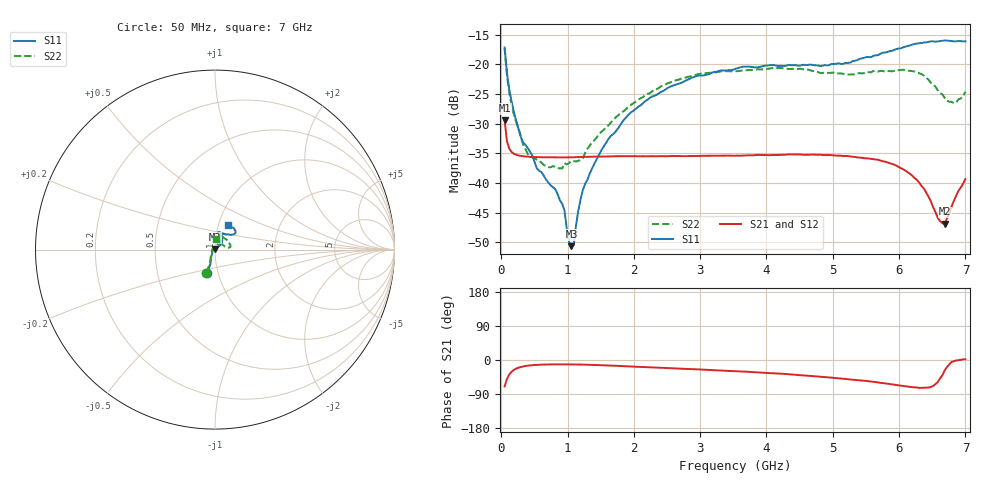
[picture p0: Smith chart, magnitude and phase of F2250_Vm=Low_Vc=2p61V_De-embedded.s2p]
! Integrated Device Technology
! Corporate Headquarters
! 6024 Silver Creek Valley Road
! San Jose, CA 95138  USA
! Phone:  1-408-284-8200
! Toll Free:  1-800-223-1366
! Webpage:  http://www.idt.com/
! Timing and RF Division
! 515 Groton Road, Suite 102
! Westford, MA 01886-6024
! Device:  F2250
! Description: Voltage Variable RF Attenuator
! Frequency:  50.0 -  6000.00 MHz
! Package:  3x3 mm Thin QFN Plastic Package: 16 pin
! Ports:  2 RF, 3 DC
!  Pin  1  = GND
!  Pin  2  = NC
!  Pin  3  = RF1  = Port 1
!  Pin  4  = NC
!  Pin  5  = GND
!  Pin  6  = GND
!  Pin  7  = GND
!  Pin  8  = GND
!  Pin  9  = NC
!  Pin 10  = RF2  = Port 2
!  Pin 11  = NC
!  Pin 12  = GND
!  Pin 13  = GND
!  Pin 14  = VCNTRL
!  Pin 15  = VDD
!  Pin 16  = VMODE
! Vcntrl:  2.610 Volts
! Vmode:  +0.000 Volts
! Vdd:  +3.30  Volts
! Current:  1.175 mA
! Data:  The device was measured on a the F2250 evaluation board which has
!  individual transmission lines to the RF pins.  Data was collected
!  using a calibrated network analyzer.  The evaluation board was
!  de-embedded using a TRL calibration technique.
!  The reference plane is the edge of the package pin.
! Misc:  SN 10
!  Action Tracker AT0258
! Date Measured:  2014-11-26
! Date:  2015-10-15  MJV
! Note:
!  Integrated Device Technology supplies this data as a sample of measured
!  data at the package pin for this product.  Your particular data for this
!  product may vary.
!  Data was taken at 25 degrees C.
!  Integrated Device Technology reserves the right to change this data at anytime.
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# GHz S dB R 50
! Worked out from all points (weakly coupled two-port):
!   201 points, 50 MHz to 7 GHz, reference 50 ohm
!   highest |S21| = -29.41 dB at 50 MHz (marker M1); lowest = -46.9 dB at 6.687 GHz (marker M2)
!   lowest |S11| = -50.6 dB at 1.058 GHz (marker M3), VSWR 1.01, Z = 49.8 + j0.245 ohm
!   |S11| at or under -10 dB: start of sweep to end of sweep
!   |S22| runs from -37.6 to -17.3 dB; largest |S21 - S12| = 4.6e-05
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0.05  -17.18 -108.6  -29.41 -69.8  -29.41 -69.8  -17.27 -111.0
0.08475  -21.45 -107.5  -32.92 -50.4  -32.92 -50.4  -21.75 -110.2
0.15425  -26.23 -116.5  -34.76 -31.1  -34.75 -31.1  -26.81 -122.4
0.29325  -32.21 -127.8  -35.43 -18.5  -35.43 -18.5  -32.10 -137.4
0.3975  -34.10 -141.8  -35.56 -15.0  -35.56 -15.0  -35.05 -160.3
0.91875  -43.49 157.8  -35.68 -11.5  -35.69 -11.5  -37.55 133.4
0.9535  -44.65 169.7  -35.69 -11.5  -35.68 -11.5  -36.66 131.1
1.023  -49.97 143.7  -35.68 -11.6  -35.68 -11.6  -36.63 116.0
1.05775  -50.63 123.2  -35.67 -11.6  -35.67 -11.6  -36.27 110.8
1.0925  -50.44 89.6  -35.66 -11.7  -35.66 -11.7  -36.30 106.4
1.162  -44.66 56.8  -35.63 -11.9  -35.64 -11.9  -36.22 95.4
1.2315  -41.10 44.2  -35.61 -12.1  -35.61 -12.1  -35.79 85.8
1.6485  -32.10 41.9  -35.52 -14.7  -35.52 -14.6  -29.88 64.6
1.96125  -28.05 42.2  -35.46 -17.2  -35.46 -17.2  -26.80 56.8
2.37825  -24.87 47.3  -35.48 -20.3  -35.48 -20.3  -23.99 56.8
3.525  -20.79 72.5  -35.40 -29.5  -35.41 -29.5  -21.19 74.7
4.7065  -20.17 72.3  -35.20 -42.5  -35.20 -42.6  -21.14 72.3
5.85325  -17.81 40.4  -36.64 -63.3  -36.64 -63.3  -21.13 23.0
6.27025  -16.51 40.0  -39.50 -72.6  -39.50 -72.7  -21.36 9.6
6.68725  -15.99 48.8  -46.86 -27.7  -46.82 -27.4  -25.64 28.5
6.861  -16.13 55.1  -42.17 -1.3  -42.13 -1.2  -26.45 58.0
7  -16.13 63.2  -39.33 1.8  -39.31 1.7  -24.62 83.2
